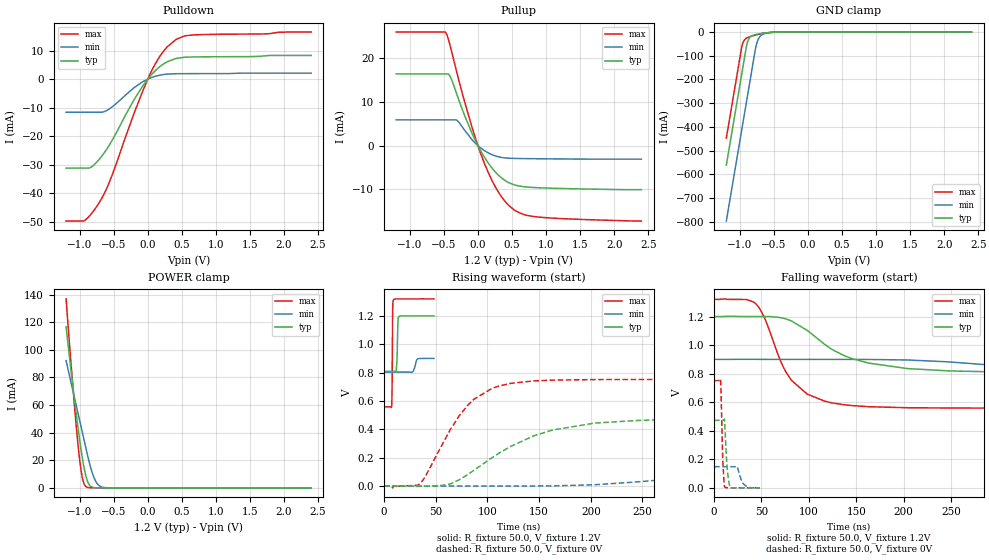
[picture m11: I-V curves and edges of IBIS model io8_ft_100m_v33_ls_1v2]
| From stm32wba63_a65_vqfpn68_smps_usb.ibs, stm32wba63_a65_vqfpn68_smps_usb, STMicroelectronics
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[Model]   io8_ft_100m_v33_ls_1v2
Model_type I/O
Polarity   Non-Inverting
Enable   Active-Low
| CAP_THRESHOLD on pad IOFT is "UDTCAPC" :
| Rising=30.0% of vddiom   Falling=70.0% of vddiom
| C_comp min and max val. don't necessarily correlate with the min and max pvt
| but are the smallest and greatest pad capacitance found.
| var   typ   min   max
C_comp   2.96668pF  2.89209pF  3.06896pF
|C_comp_pullup   1.71350pF  1.55617pF  1.85262pF
|C_comp_pulldown   1.25318pF  1.33592pF  1.21634pF
Vinl = 450.0mV
Vinh = 660.0mV
Vmeas = 600.0mV   | Reference voltage for timing measurements
Cref  = 50.0pF   | Timing specification test load capacitance value
Rref  = 1.0MOhm   | Timing specification test load resistance value
Vref  = 660.0mV   | Timing specification test load voltage
[Model Spec]
| TIME_THRESHOLD on pin ZIV33M is "CMOS" :
| Rising=50.0% of vddiom   Falling=50.0% of vddiom
Vinl 436.50000mV 331.50000mV 482.50000mV
Vinh 753.50000mV 549.50000mV 837.50000mV
| variable   typ   min   max
[Temperature Range] 25.0 140.0 -40.0
| variable   typ   min   max
[Voltage Range] 1.2V 900.0mV 1.32V
| variable   typ   min   max
[POWER Clamp Reference] 1.2V 900.0mV 1.32V
| variable   typ   min   max
[GND Clamp Reference] 0V 0V 0V
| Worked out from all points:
|   slope of the pulldown table from 0 to 0.18 V, typ, clamps not added: 40.6 ohm
|   slope of the pullup table from 0 to 0.18 V, typ, clamps not added: 39.4 ohm
|   GND clamp passes 1 mA (typ) near -0.51 V on its own axis
|   POWER clamp passes 1 mA (typ) near -0.83 V on its own axis
|   rising waveform, R_fixture 50.0, V_fixture 1.2V: 20-80 % time 818ps typ, 2.2ns min, 432ps max; typ from 0.809 V to 1.2 V
|   falling waveform, R_fixture 50.0, V_fixture 1.2V: 20-80 % time 62.1ns typ, 155ns min, 34.3ns max; typ from 1.2 V to 0.809 V
|   rising waveform, R_fixture 50.0, V_fixture 0V: 20-80 % time 72ns typ, 179ns min, 39.5ns max; typ from 0 V to 0.473 V
|   falling waveform, R_fixture 50.0, V_fixture 0V: 20-80 % time 2.69ns typ, 5.05ns min, 1.94ns max; typ from 0.473 V to 0 V
[POWER Clamp]
-1.2V     116.7mA    92.13mA    136.9mA
-1.09V    69.42mA    68.21mA    67.14mA
-1.02V    41.75mA    52.99mA    28.91mA
-990mV    30.98mA    46.47mA    16.09mA
-970mV    24.36mA    42.12mA    9.575mA
-940mV    15.59mA    35.6mA     3.485mA
-910mV    8.693mA    29.07mA    1.01mA
-860mV    2.259mA    18.59mA    104.6uA
-780mV    143.1uA    6.246mA    2.555uA
-720mV    16.22uA    1.846mA    157.1nA
-650mV    1.267uA    330.3uA    6.118nA
2.4V      0A         0A         0A
[GND Clamp]
-1.2V     -561.6mA   -797.4mA   -447.4mA
-980mV    -187.6mA   -423.4mA   -73.43mA
-960mV    -153.6mA   -389.4mA   -48.26mA
-900mV    -54.17mA   -287.4mA   -24.97mA
-870mV    -29.55mA   -236.4mA   -21.19mA
-830mV    -17.05mA   -168.4mA   -17.42mA
-760mV    -9.921mA   -54.55mA   -11.89mA
-730mV    -8.191mA   -29.78mA   -9.811mA
-690mV    -6.26mA    -14.49mA   -7.318mA
-600mV    -2.976mA   -4.315mA   -3.058mA
-380mV    -57.63uA   -251uA     -19.49uA
2.4V      872.7pA    204.8nA    349.4pA
| variable   typ   min   max
[Pullup Reference] 1.2V 900.0mV 1.32V
| variable   typ   min   max
[Pulldown Reference] 0V 0V 0V
[Pullup]
-1.2V     16.39mA    5.903mA    25.96mA
-470mV    16.39mA    5.903mA    25.8mA
-410mV    15.89mA    5.903mA    22.96mA
-310mV    11.76mA    5.823mA    16.75mA
-80mV     2.58mA     1.232mA    3.849mA
80mV      -2.237mA   -962.6uA   -3.434mA
190mV     -4.777mA   -1.94mA    -7.418mA
310mV     -6.857mA   -2.571mA   -10.82mA
540mV     -8.979mA   -2.91mA    -14.76mA
670mV     -9.371mA   -2.949mA   -15.71mA
920mV     -9.627mA   -2.991mA   -16.35mA
2.4V      -10.04mA   -3.075mA   -17.21mA
[Pulldown]
-1.2V     -31.2mA    -11.62mA   -49.78mA
-930mV    -31.2mA    -11.62mA   -49.64mA
-830mV    -30.86mA   -11.62mA   -47.25mA
-710mV    -28.04mA   -11.62mA   -43.19mA
-550mV    -22.55mA   -10.2mA    -35.3mA
-200mV    -7.146mA   -2.964mA   -11.89mA
40mV      1.171mA    405.8uA    2.092mA
130mV     3.416mA    1.118mA    6.182mA
230mV     5.302mA    1.613mA    9.763mA
420mV     7.288mA    1.898mA    13.99mA
670mV     7.779mA    1.924mA    15.51mA
2.4V      8.319mA    2.102mA    16.52mA
[Ramp]
dV/dt_r 283.7937mV/71.05404ns 88.92894mV/177.1903ns 450.9923mV/39.13006ns
dV/dt_f 234.65962mV/60.35006ns 57.89322mV/154.89549ns 456.73577mV/32.74659ns
R_load = 50.0
| Removed startup time: 0s 0s 0s  .
| Removed end time: 48.35ns.
[Rising Waveform]
R_fixture   = 50.0
V_fixture   = 1.2V
V_fixture_min = 900.0mV
V_fixture_max = 1.32V
0s        808.9mV    803.5mV    558.8mV
7.4ns     808.9mV    803.5mV    557.2mV
7.9ns     808.9mV    803.5mV    718.4mV
8.4ns     808.9mV    803.5mV    1.224V
8.9ns     808.9mV    803.5mV    1.308V
11.85ns   805.5mV    803.5mV    1.319V
12.65ns   898mV      803.5mV    1.319V
13.6ns    1.166V     803.5mV    1.319V
14.8ns    1.197V     803.5mV    1.32V
48.35ns   1.2V       899.9mV    1.32V
| Removed startup time: 0s 0s 0s  .
| Removed end time: 1.998us.
[Falling Waveform]
R_fixture   = 50.0
V_fixture   = 1.2V
V_fixture_min = 900.0mV
V_fixture_max = 1.32V
0s        1.2V       900mV      1.32V
44.5ns    1.2V       900.3mV    1.286V
53.75ns   1.2V       900.1mV    1.181V
75.5ns    1.184V     900mV      814.4mV
98.25ns   1.103V     900mV      656.5mV
124.5ns   969.3mV    900mV      595.2mV
163ns     873.9mV    899.3mV    568.5mV
260ns     817.3mV    876.4mV    559.1mV
530.3ns   808.9mV    810.1mV    558.8mV
1.998us   808.9mV    803.5mV    558.8mV
| Removed startup time: 0s 0s 0s  .
| Removed end time: 1.998us.
[Rising Waveform]
R_fixture   = 50.0
V_fixture   = 0V
V_fixture_min = 0V
V_fixture_max = 0V
0s        4.821nV    215.5nV    3.377nV
34.75ns   -112.3uV   -401.2uV   17.33mV
63.75ns   13.28mV    -25.65uV   393.1mV
87.25ns   112.4mV    -9.499uV   613.3mV
111.5ns   232.8mV    65.96uV    705.9mV
144.5ns   353.1mV    477.5uV    741.1mV
244.8ns   462.2mV    29.24mV    751.4mV
396.8ns   472.5mV    110.6mV    751.6mV
571ns     472.9mV    141.5mV    751.6mV
1.998us   473mV      148.2mV    751.7mV
| Removed startup time: 0s 0s 0s  .
| Removed end time: 48.35ns.
[Falling Waveform]
R_fixture   = 50.0
V_fixture   = 0V
V_fixture_min = 0V
V_fixture_max = 0V
0s        473mV      148.3mV    751.7mV
6.9ns     473mV      148.3mV    757.3mV
9.1ns     473mV      148.3mV    212.4mV
11.15ns   461.4mV    148.3mV    6.931mV
13.85ns   130.5mV    148.3mV    882.9uV
16.8ns    5.455mV    148.3mV    278.1uV
23.95ns   180.6uV    152.3mV    165.8uV
29.65ns   88.75uV    41.14mV    171.6uV
34.55ns   81.01uV    8.713mV    202.9uV
48.35ns   86.46uV    191.3uV    193.1uV
